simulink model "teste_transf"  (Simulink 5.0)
settings: Solver=ode5  StartTime=0.0  StopTime=100  FixedStep=0.002  RelTol=1e-3
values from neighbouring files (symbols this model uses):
  Apr = 5.249    [dados_19_2.m]
  cp = 0.12    [dados_19_2.m]
  cPr = 1.0    (= 1)    [dados_19_2.m]
  rho = 800.92    [dados_19_2.m]
  rhop = 8201.5    [dados_19_2.m]
  T0 = 25    [dados_19_2.m]
  Tlim = 93    [dados_19_2.m]
  Tp0 = 25    [dados_19_2.m]
  Uap = 32.550    (= 32.55)    [dados_19_2.m]
  Upr = 13.020    (= 13.02)    [dados_19_2.m]
  Uvp = 81.374    [dados_19_2.m]
  V = 1.2035    [dados_19_2.m]
  Vp = 0.2667    [dados_19_2.m]
undefined symbols (not defined in the file or in its folder): Acam

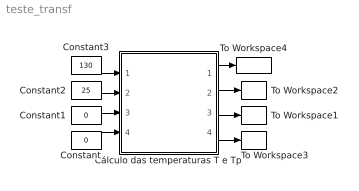
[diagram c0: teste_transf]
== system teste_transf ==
  Constant : Constant  Value=0
  Constant1 : Constant  Value=0
  Constant2 : Constant  Value=25
  Constant3 : Constant  Value=130
  Cálculo das temperaturas T e Tp : Subsystem
  To Workspace1 : ToWorkspace  VariableName=qap  SampleTime=-1  SaveFormat=Array
  To Workspace2 : ToWorkspace  VariableName=qvp  SampleTime=-1  SaveFormat=Array
  To Workspace3 : ToWorkspace  VariableName=T  SampleTime=-1  SaveFormat=Array
  To Workspace4 : ToWorkspace  VariableName=Chav  SampleTime=-1  SaveFormat=Array
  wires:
  Constant/1 -> Cálculo das temperaturas T e Tp/4(q2)
  Constant1/1 -> Cálculo das temperaturas T e Tp/3(q1)
  Constant2/1 -> Cálculo das temperaturas T e Tp/2(Ta)
  Constant3/1 -> Cálculo das temperaturas T e Tp/1(Tv)
  Cálculo das temperaturas T e Tp/2(qvp) -> To Workspace2/1
  Cálculo das temperaturas T e Tp/3(qap) -> To Workspace1/1
  Cálculo das temperaturas T e Tp/4(T) -> To Workspace3/1
  Cálculo das temperaturas T e Tp/1(Chav) -> To Workspace4/1

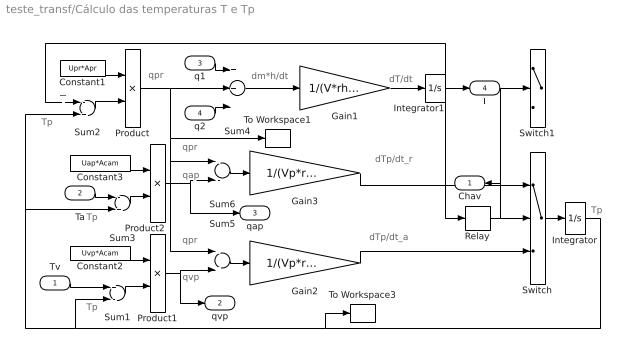
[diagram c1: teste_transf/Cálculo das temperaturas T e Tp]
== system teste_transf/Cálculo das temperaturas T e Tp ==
  note: Tp
  note: qpr
  note: Tp
  note: qvp
  note: Tp
  note: qap
  note: dm*h/dt
  note: dT/dt
  note: T
  note: dTp/dt_r
  note: dTp/dt_a
  note: qpr
  note: qpr
  note: Tp
  Tv : Inport
  Ta : Inport  Port=2
  q1 : Inport  Port=3
  q2 : Inport  Port=4
  Constant1 : Constant  Value=Upr*Apr
  Constant2 : Constant  Value=Uvp*Acam
  Constant3 : Constant  Value=Uap*Acam
  Gain1 : Gain  Gain=1/(V*rho*cPr)
  Gain2 : Gain  Gain=1/(Vp*rhop*cp)
  Gain3 : Gain  Gain=1/(Vp*rhop*cp)
  Integrator : Integrator  InitialCondition=Tp0
  Integrator1 : Integrator  InitialCondition=T0
  Product : Product
  Product1 : Product
  Product2 : Product
  Relay : Relay  OnSwitchValue=Tlim  OffSwitchValue=T0
  Sum1 : Sum  Inputs=+-
  Sum2 : Sum  Inputs=-+
  Sum3 : Sum  Inputs=-+
  Sum4 : Sum  Inputs=3
  Sum5 : Sum  Inputs=-+
  Sum6 : Sum  Inputs=--
  Switch : Switch  Threshold=0.5
  Switch1 : Switch  Threshold=0.5
  To Workspace1 : ToWorkspace  VariableName=qpr  SampleTime=-1  SaveFormat=Array
  To Workspace3 : ToWorkspace  VariableName=Tp  SampleTime=-1  SaveFormat=Array
  Chav : Outport  Orientation=left
  qvp : Outport  Port=2
  qap : Outport  Port=3
  T : Outport  Port=4
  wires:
  Sum2/1 -> Product/2
  Constant1/1 -> Product/1
  Product/1 -> Sum4/2, Sum6/1, Sum5/1, To Workspace1/1
  Tv/1 -> Sum1/1
  Constant2/1 -> Product1/1
  Product1/1 -> Sum5/2, qvp/1
  Ta/1 -> Sum3/1
  Constant3/1 -> Product2/1
  Product2/1 -> Sum6/2, qap/1
  q2/1 -> Sum4/3
  q1/1 -> Sum4/1
  Sum4/1 -> Gain1/1
  Gain1/1 -> Integrator1/1
  Integrator1/1 -> Sum2/1, Relay/1, T/1
  Sum5/1 -> Gain2/1
  Gain2/1 -> Switch/3
  Sum6/1 -> Gain3/1
  Relay/1 -> Switch/2, Chav/1, Switch1/2
  Gain3/1 -> Switch/1
  Switch/1 -> Integrator/1
  Sum1/1 -> Product1/2
  Integrator/1 -> Sum1/2, Sum3/2, Sum2/2, To Workspace3/1
  Sum3/1 -> Product2/2
